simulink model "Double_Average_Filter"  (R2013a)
settings: Solver=FixedStepDiscrete  SolverMode=SingleTasking  StartTime=0.0  StopTime=inf  FixedStep=Ts  RelTol=1e-3
PreLoadFcn:
  | Implementation_Settings
StartFcn:
  | Implementation_Settings
undefined symbols (not defined in the file or in its folder): Channel, hex2dec, OffsetVolt, OutputChannel
libraries: opcode x20, pec x11

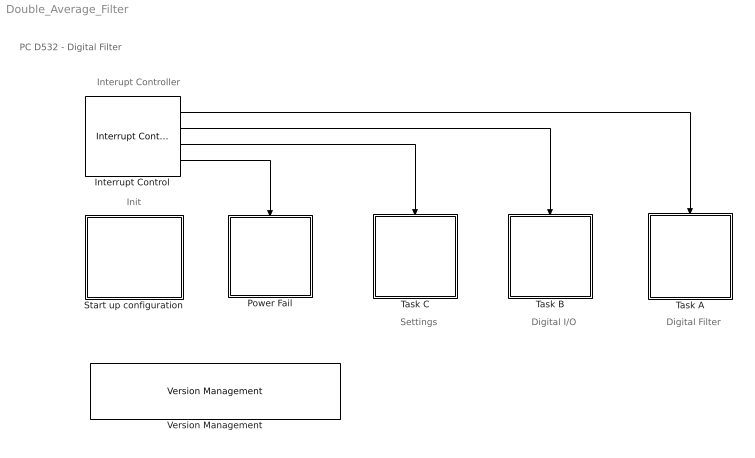
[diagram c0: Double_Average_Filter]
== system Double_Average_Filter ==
  note: PC D532 - Digital Filter
  note: Digital Filter
  note: Interupt Controller
  note: Digital I/O
  note: Settings
  note: Init
  Interrupt Control : pec/Tasks/Interrupt Control  Tag=AsyncRateTransition  EN_A=on  EN_B=on  EN_C=on  ct=Base_cycle_time  k1=Task_A_mult  k2=Task_B_mult  k3=Task_C_mult
  Power Fail : Subsystem  TreatAsAtomicUnit=on
  Start up configuration : Subsystem
  Task A : Subsystem  TreatAsAtomicUnit=on
  Task B : Subsystem  TreatAsAtomicUnit=on
  Task C : Subsystem  TreatAsAtomicUnit=on
  Version Management : pec/Logo, Info/Version Management  ApplDescr='Digital Filter'  ApplVersion='1.0.0.0'  OutPortVisible=off
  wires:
  Interrupt Control/4 -> Power Fail/Trigger
  Interrupt Control/2 -> Task B/Trigger
  Interrupt Control/3 -> Task C/Trigger
  Interrupt Control/1 -> Task A/Trigger

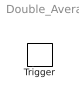
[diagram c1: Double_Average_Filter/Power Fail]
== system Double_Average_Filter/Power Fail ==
  Trigger : TriggerPort  TriggerType=function-call

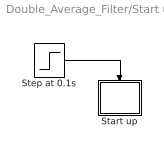
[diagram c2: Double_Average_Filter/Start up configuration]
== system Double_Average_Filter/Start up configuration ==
  Start up : Subsystem  TreatAsAtomicUnit=on
  Step at 0.1s : Step  Time=0.1  SampleTime=0
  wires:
  Step at 0.1s/1 -> Start up/Trigger

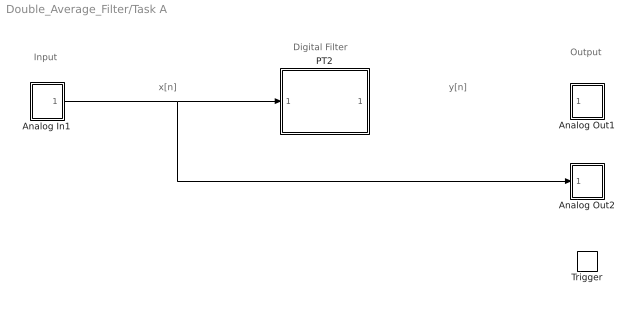
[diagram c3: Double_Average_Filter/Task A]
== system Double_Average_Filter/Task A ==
  note: Input
  note: Output
  note: Digital Filter
  note: y[n]
  note: x[n]
  Trigger : TriggerPort  TriggerType=function-call
  Analog In1 : Subsystem
  Analog Out1 : Subsystem
  Analog Out2 : Subsystem
  PT2 : Subsystem  TreatAsAtomicUnit=on
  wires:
  Analog In1/1(Out) -> PT2/1(y_in), Analog Out2/1(In1)
  ? -> Analog Out1/1(In1)

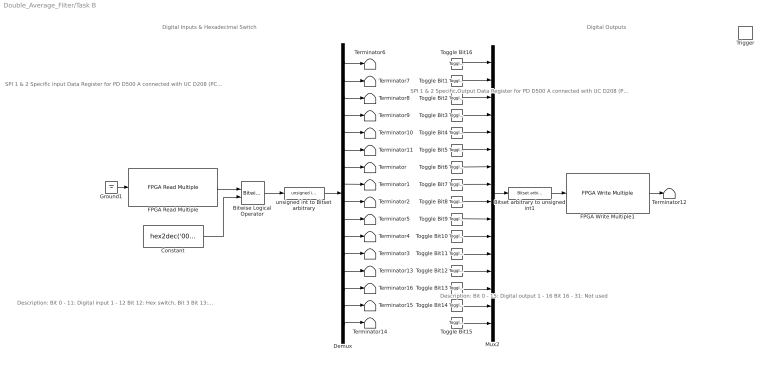
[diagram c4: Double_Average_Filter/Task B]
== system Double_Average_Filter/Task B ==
  note: Digital Inputs & Hexadecimal Switch
  note: Digital Outputs
  note: Description: Bit 0 - 15: Digital output 1 - 16 Bit 16 - 31: Not used
  note: SPI 1 & 2 Specific Output Data Register for PD D500 A connected with UC D208 (PC D532) Type: DPRAM Array 1 (32bit ports) Address offset: 0x07C000 Adress: 0x008 Mode: Write
  note: Description: Bit 0 - 11: Digital input 1 - 12 Bit 12: Hex switch, Bit 3 Bit 13: Hex switch, Bit 2 Bit 14: Hex switch, Bit 1 Bit 15: Hex switch, Bit 0 Bit 16 - 31: Not used
  note: SPI 1 & 2 Specific Input Data Register for PD D500 A connected with UC D208 (PC D532) Type: DPRAM Array 1 (32bit ports) Address offset: 0x05C000 Adress: 0x008 Mode: Read
  Trigger : TriggerPort  TriggerType=function-call
  Bitset arbitrary to unsigned int1 : opcode/Binary Signals/Bitset arbitrary to unsigned int  in_width=16  OutDataType=uint32
  Bitwise Logical Operator : pec/Math/Bitwise Logical Operator  Operator=XOR
  Constant : Constant  Value=hex2dec('00000FFF')  OutDataTypeStr=uint32
  Demux : Demux  Outputs=16
  FPGA Read Multiple : pec/Sources/FPGA Read Multiple  AddrOffsetHex=hex2dec('05c008')  number=1  datatype=uint32  pciBusPop=0  barPop=0
  FPGA Write Multiple1 : pec/Sinks/FPGA Write Multiple  AddrOffsetHex=hex2dec('07C008')  number=1  enaWriteProt=off  pciBusPop=0  barPop=0
  Ground1 : Ground
  Mux2 : Mux  Inputs=16
  Terminator{,1..16} (17 alike) : Terminator
  Toggle Bit{1..16} (16 alike) : opcode/Sources/Toggle Bit  xBit=0
  unsigned int to Bitset arbitrary : opcode/Binary Signals/unsigned int to Bitset arbitrary  InDataType=uint32  out_width=16
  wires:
  Toggle Bit2/1 -> Mux2/3
  Toggle Bit1/1 -> Mux2/2
  Toggle Bit16/1 -> Mux2/1
  Toggle Bit3/1 -> Mux2/4
  Toggle Bit4/1 -> Mux2/5
  Toggle Bit5/1 -> Mux2/6
  Toggle Bit6/1 -> Mux2/7
  Toggle Bit7/1 -> Mux2/8
  Toggle Bit8/1 -> Mux2/9
  Toggle Bit9/1 -> Mux2/10
  Toggle Bit10/1 -> Mux2/11
  Toggle Bit11/1 -> Mux2/12
  Toggle Bit12/1 -> Mux2/13
  Toggle Bit13/1 -> Mux2/14
  Toggle Bit14/1 -> Mux2/15
  Toggle Bit15/1 -> Mux2/16
  Bitset arbitrary to unsigned int1/1 -> FPGA Write Multiple1/1
  FPGA Write Multiple1/1 -> Terminator12/1
  Mux2/1 -> Bitset arbitrary to unsigned int1/1
  Demux/16 -> Terminator14/1
  Demux/15 -> Terminator15/1
  Demux/14 -> Terminator16/1
  Demux/13 -> Terminator13/1
  unsigned int to Bitset arbitrary/1 -> Demux/1
  Demux/1 -> Terminator6/1
  Demux/2 -> Terminator7/1
  Demux/3 -> Terminator8/1
  Demux/4 -> Terminator9/1
  Demux/5 -> Terminator10/1
  Demux/6 -> Terminator11/1
  Demux/7 -> Terminator/1
  Demux/8 -> Terminator1/1
  Demux/9 -> Terminator2/1
  Demux/10 -> Terminator5/1
  Demux/11 -> Terminator4/1
  Demux/12 -> Terminator3/1
  Bitwise Logical Operator/1 -> unsigned int to Bitset arbitrary/1
  Constant/1 -> Bitwise Logical Operator/2
  Ground1/1 -> FPGA Read Multiple/1
  FPGA Read Multiple/1 -> Bitwise Logical Operator/1

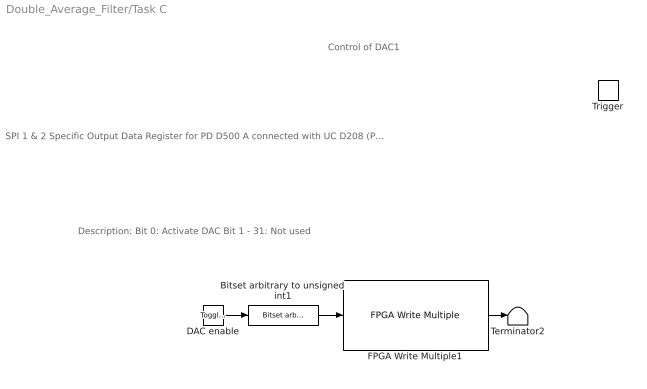
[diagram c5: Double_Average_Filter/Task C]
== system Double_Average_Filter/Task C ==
  note: SPI 1 & 2 Specific Output Data Register for PD D500 A connected with UC D208 (PC D532) Type: DPRAM Array 1 (32bit ports) Address offset: 0x07C000 Adress: 0x00C Mode: Write
  note: Description: Bit 0: Activate DAC Bit 1 - 31: Not used
  note: Control of DAC1
  Trigger : TriggerPort  TriggerType=function-call
  Bitset arbitrary to unsigned int1 : opcode/Binary Signals/Bitset arbitrary to unsigned int  in_width=1  OutDataType=uint32
  DAC enable : opcode/Sources/Toggle Bit  xBit=1
  FPGA Write Multiple1 : pec/Sinks/FPGA Write Multiple  AddrOffsetHex=hex2dec('07C00C')  number=1  enaWriteProt=off  pciBusPop=0  barPop=0
  Terminator2 : Terminator
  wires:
  Bitset arbitrary to unsigned int1/1 -> FPGA Write Multiple1/1
  DAC enable/1 -> Bitset arbitrary to unsigned int1/1
  FPGA Write Multiple1/1 -> Terminator2/1

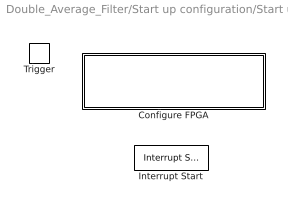
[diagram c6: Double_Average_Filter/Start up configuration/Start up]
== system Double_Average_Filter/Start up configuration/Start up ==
  Trigger : TriggerPort
  Configure FPGA : Subsystem  Priority=1
  Interrupt Start : pec/Tasks/Interrupt Start  Priority=1000

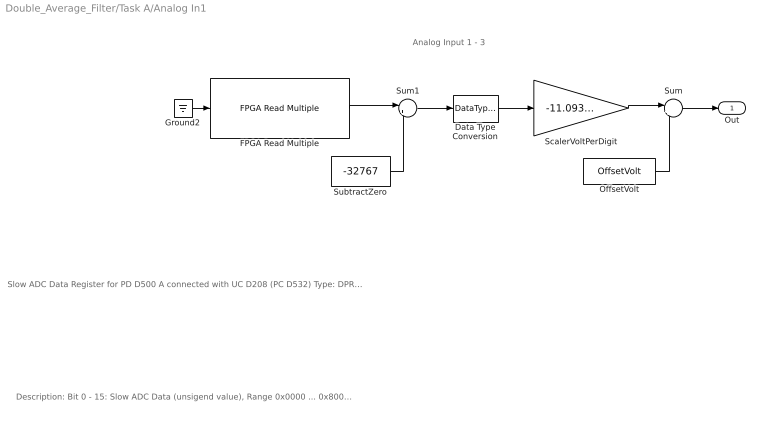
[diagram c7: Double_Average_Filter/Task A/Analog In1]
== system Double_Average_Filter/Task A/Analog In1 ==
  note: Analog Input 1 - 3
  note: Description: Bit 0 - 15: Slow ADC Data (unsigend value), Range 0x0000 ... 0x8000 ... 0xFFFF is +11.0939V ... 0 ... -11.0939V Bit 16 - 31: Not used
  note: Slow ADC Data Register for PD D500 A connected with UC D208 (PC D532) Type: DPRAM Array 1 (32bit ports) Address: 0x05C800 Address offset: 0x018 (Channel 7 - Analog Input 1) 0x01C (Channel 8 - Analog Input 2) 0x020 (Channel 9 - Analog Input 3) Mode: Read
  Data Type Conversion : DataTypeConversion  OutDataTypeStr=double
  FPGA Read Multiple : pec/Sources/FPGA Read Multiple  AddrOffsetHex=hex2dec('05c800') + 4*((Channel-1) + 6)  number=1  datatype=int32  pciBusPop=0  barPop=0
  Ground2 : Ground
  OffsetVolt : Constant  Value=OffsetVolt
  ScalerVoltPerDigit : Gain  Gain=-11.0939/32767
  SubtractZero : Constant  Value=-32767  OutDataTypeStr=int32
  Sum : Sum  Inputs=|++
  Sum1 : Sum  Inputs=|++
  Out : Outport
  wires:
  OffsetVolt/1 -> Sum/2
  Data Type Conversion/1 -> ScalerVoltPerDigit/1
  ScalerVoltPerDigit/1 -> Sum/1
  Sum/1 -> Out/1
  FPGA Read Multiple/1 -> Sum1/1
  SubtractZero/1 -> Sum1/2
  Sum1/1 -> Data Type Conversion/1
  Ground2/1 -> FPGA Read Multiple/1

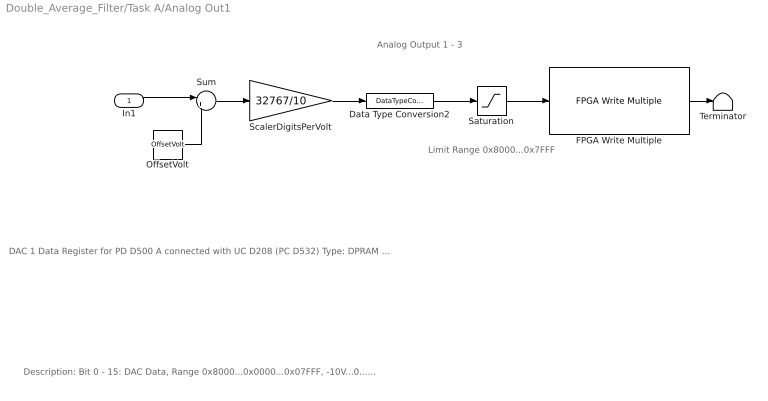
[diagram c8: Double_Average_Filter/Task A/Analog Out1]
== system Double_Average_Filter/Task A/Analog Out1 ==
  note: Limit Range 0x8000...0x7FFF
  note: DAC 1 Data Register for PD D500 A connected with UC D208 (PC D532) Type: DPRAM Array 1 (32bit ports) Address offset: 0x07C800 Adress: 0x000 (Channel 1), 0x004 (Channel 2), 0x008 (Channel 3) Mode: Write
  note: Description: Bit 0 - 15: DAC Data, Range 0x8000...0x0000...0x07FFF, -10V...0...10V, Resolution 10V/2^15 Bit 16 - 31: Not used
  note: Analog Output 1 - 3
  In1 : Inport
  Data Type Conversion2 : DataTypeConversion  OutDataTypeStr=int32
  FPGA Write Multiple : pec/Sinks/FPGA Write Multiple  AddrOffsetHex=hex2dec('07C800') + 4*(OutputChannel-1)  number=1  enaWriteProt=off  pciBusPop=0  barPop=0
  OffsetVolt : Constant  Value=OffsetVolt
  Saturation : Saturate  UpperLimit=32767  LowerLimit=-32767
  ScalerDigitsPerVolt : Gain  Gain=32767/10
  Sum : Sum  Inputs=|++
  Terminator : Terminator
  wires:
  Saturation/1 -> FPGA Write Multiple/1
  Data Type Conversion2/1 -> Saturation/1
  ScalerDigitsPerVolt/1 -> Data Type Conversion2/1
  Sum/1 -> ScalerDigitsPerVolt/1
  OffsetVolt/1 -> Sum/2
  In1/1 -> Sum/1
  FPGA Write Multiple/1 -> Terminator/1

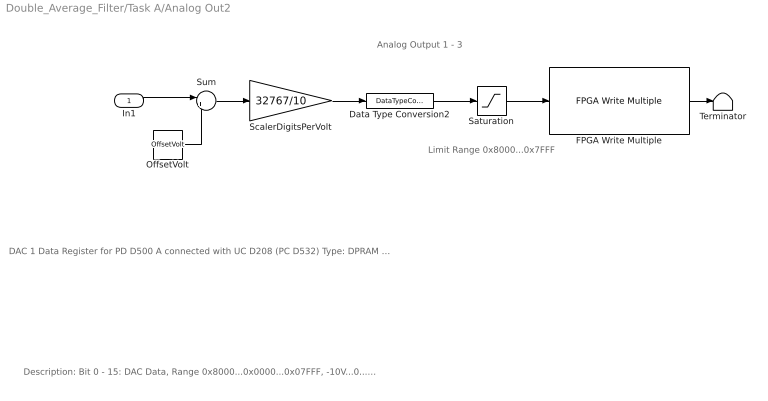
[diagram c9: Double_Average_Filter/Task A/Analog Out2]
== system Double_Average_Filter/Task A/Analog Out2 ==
  note: Analog Output 1 - 3
  note: Description: Bit 0 - 15: DAC Data, Range 0x8000...0x0000...0x07FFF, -10V...0...10V, Resolution 10V/2^15 Bit 16 - 31: Not used
  note: DAC 1 Data Register for PD D500 A connected with UC D208 (PC D532) Type: DPRAM Array 1 (32bit ports) Address offset: 0x07C800 Adress: 0x000 (Channel 1), 0x004 (Channel 2), 0x008 (Channel 3) Mode: Write
  note: Limit Range 0x8000...0x7FFF
  In1 : Inport
  Data Type Conversion2 : DataTypeConversion  OutDataTypeStr=int32
  FPGA Write Multiple : pec/Sinks/FPGA Write Multiple  AddrOffsetHex=hex2dec('07C800') + 4*(OutputChannel-1)  number=1  enaWriteProt=off  pciBusPop=0  barPop=0
  OffsetVolt : Constant  Value=OffsetVolt
  Saturation : Saturate  UpperLimit=32767  LowerLimit=-32767
  ScalerDigitsPerVolt : Gain  Gain=32767/10
  Sum : Sum  Inputs=|++
  Terminator : Terminator
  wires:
  FPGA Write Multiple/1 -> Terminator/1
  In1/1 -> Sum/1
  OffsetVolt/1 -> Sum/2
  Sum/1 -> ScalerDigitsPerVolt/1
  ScalerDigitsPerVolt/1 -> Data Type Conversion2/1
  Data Type Conversion2/1 -> Saturation/1
  Saturation/1 -> FPGA Write Multiple/1

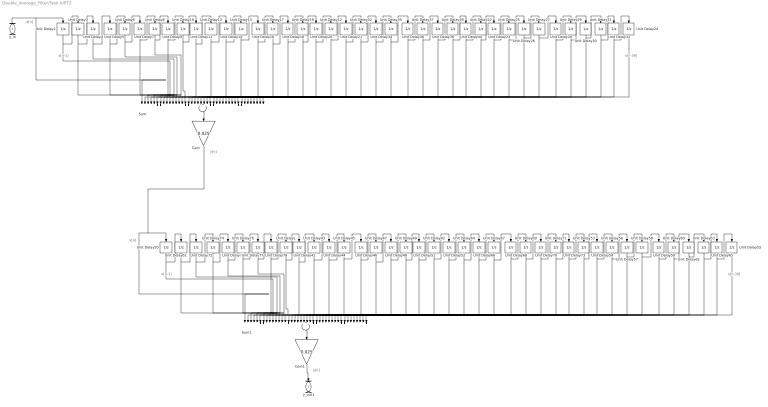
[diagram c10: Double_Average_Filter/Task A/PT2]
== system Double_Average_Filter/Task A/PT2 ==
  note: x[n]
  note: x[n-39]
  note: y[n]
  note: x[n-1]
  note: x[n]
  note: x[n-39]
  note: y[n]
  note: x[n-1]
  y_in : Inport
  Gain : Gain  Gain=0.025
  Gain1 : Gain  Gain=0.025
  Sum : Sum  Inputs=++++++++++++++++++++++++++++++++++++++++
  Sum1 : Sum  Inputs=++++++++++++++++++++++++++++++++++++++++
  Unit Delay{1..78} (78 alike) : UnitDelay  SampleTime=-1
  y_out1 : Outport
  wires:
  Sum/1 -> Gain/1
  Unit Delay2/1 -> Sum/2, Unit Delay3/1
  Unit Delay3/1 -> Sum/3, Unit Delay4/1
  Unit Delay4/1 -> Sum/4, Unit Delay5/1
  Unit Delay5/1 -> Sum/5, Unit Delay6/1
  Unit Delay6/1 -> Sum/6, Unit Delay7/1
  Unit Delay7/1 -> Sum/7, Unit Delay8/1
  Unit Delay8/1 -> Sum/8, Unit Delay9/1
  Unit Delay9/1 -> Sum/9, Unit Delay10/1
  Unit Delay10/1 -> Sum/10, Unit Delay11/1
  Unit Delay11/1 -> Sum/11, Unit Delay13/1
  Unit Delay13/1 -> Sum/12, Unit Delay14/1
  Unit Delay14/1 -> Sum/13, Unit Delay15/1
  Unit Delay15/1 -> Sum/14, Unit Delay16/1
  Unit Delay16/1 -> Sum/15, Unit Delay17/1
  Unit Delay17/1 -> Sum/16, Unit Delay18/1
  Unit Delay18/1 -> Sum/17, Unit Delay19/1
  Unit Delay19/1 -> Sum/18, Unit Delay20/1
  Unit Delay20/1 -> Sum/19, Unit Delay12/1
  Unit Delay12/1 -> Sum/20, Unit Delay21/1
  Unit Delay21/1 -> Sum/21, Unit Delay32/1
  Unit Delay32/1 -> Sum/22, Unit Delay34/1
  Unit Delay34/1 -> Sum/23, Unit Delay35/1
  Unit Delay35/1 -> Sum/24, Unit Delay36/1
  Unit Delay36/1 -> Sum/25, Unit Delay37/1
  Unit Delay37/1 -> Sum/26, Unit Delay38/1
  Unit Delay38/1 -> Sum/27, Unit Delay39/1
  Unit Delay39/1 -> Sum/28, Unit Delay40/1
  Unit Delay40/1 -> Sum/29, Unit Delay22/1
  Unit Delay22/1 -> Sum/30, Unit Delay23/1
  Unit Delay23/1 -> Sum/31, Unit Delay25/1
  Unit Delay25/1 -> Sum/32, Unit Delay26/1
  Unit Delay26/1 -> Sum/33, Unit Delay27/1
  Unit Delay27/1 -> Sum/34, Unit Delay28/1
  Unit Delay28/1 -> Sum/35, Unit Delay29/1
  Unit Delay29/1 -> Sum/36, Unit Delay30/1
  Unit Delay30/1 -> Sum/37, Unit Delay31/1
  Unit Delay31/1 -> Sum/38, Unit Delay33/1
  Unit Delay33/1 -> Sum/39, Unit Delay24/1
  Unit Delay24/1 -> Sum/40
  y_in/1 -> Unit Delay2/1, Sum/1
  Gain1/1 -> y_out1/1
  Sum1/1 -> Gain1/1
  Unit Delay50/1 -> Sum1/2, Unit Delay61/1
  Unit Delay61/1 -> Sum1/3, Unit Delay72/1
  Unit Delay72/1 -> Sum1/4, Unit Delay74/1
  Unit Delay74/1 -> Sum1/5, Unit Delay75/1
  Unit Delay75/1 -> Sum1/6, Unit Delay76/1
  Unit Delay76/1 -> Sum1/7, Unit Delay77/1
  Unit Delay77/1 -> Sum1/8, Unit Delay78/1
  Unit Delay78/1 -> Sum1/9, Unit Delay1/1
  Unit Delay1/1 -> Sum1/10, Unit Delay41/1
  Unit Delay41/1 -> Sum1/11, Unit Delay43/1
  Unit Delay43/1 -> Sum1/12, Unit Delay44/1
  Unit Delay44/1 -> Sum1/13, Unit Delay45/1
  Unit Delay45/1 -> Sum1/14, Unit Delay46/1
  Unit Delay46/1 -> Sum1/15, Unit Delay47/1
  Unit Delay47/1 -> Sum1/16, Unit Delay48/1
  Unit Delay48/1 -> Sum1/17, Unit Delay49/1
  Unit Delay49/1 -> Sum1/18, Unit Delay51/1
  Unit Delay51/1 -> Sum1/19, Unit Delay42/1
  Unit Delay42/1 -> Sum1/20, Unit Delay52/1
  Unit Delay52/1 -> Sum1/21, Unit Delay64/1
  Unit Delay64/1 -> Sum1/22, Unit Delay66/1
  Unit Delay66/1 -> Sum1/23, Unit Delay67/1
  Unit Delay67/1 -> Sum1/24, Unit Delay68/1
  Unit Delay68/1 -> Sum1/25, Unit Delay69/1
  Unit Delay69/1 -> Sum1/26, Unit Delay70/1
  Unit Delay70/1 -> Sum1/27, Unit Delay71/1
  Unit Delay71/1 -> Sum1/28, Unit Delay73/1
  Unit Delay73/1 -> Sum1/29, Unit Delay53/1
  Unit Delay53/1 -> Sum1/30, Unit Delay54/1
  Unit Delay54/1 -> Sum1/31, Unit Delay56/1
  Unit Delay56/1 -> Sum1/32, Unit Delay57/1
  Unit Delay57/1 -> Sum1/33, Unit Delay58/1
  Unit Delay58/1 -> Sum1/34, Unit Delay59/1
  Unit Delay59/1 -> Sum1/35, Unit Delay60/1
  Unit Delay60/1 -> Sum1/36, Unit Delay62/1
  Unit Delay62/1 -> Sum1/37, Unit Delay63/1
  Unit Delay63/1 -> Sum1/38, Unit Delay65/1
  Unit Delay65/1 -> Sum1/39, Unit Delay55/1
  Unit Delay55/1 -> Sum1/40
  Gain/1 -> Sum1/1, Unit Delay50/1

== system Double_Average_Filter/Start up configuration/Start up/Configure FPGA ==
  For Iterator Subsystem : Subsystem  TreatAsAtomicUnit=on

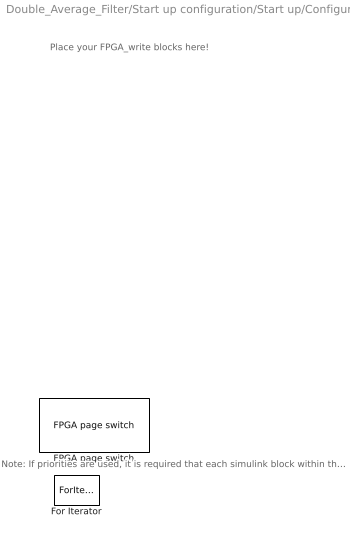
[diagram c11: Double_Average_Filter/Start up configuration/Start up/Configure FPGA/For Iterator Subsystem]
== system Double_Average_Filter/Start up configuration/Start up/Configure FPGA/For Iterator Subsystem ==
  note: Place your FPGA_write blocks here!
  note: Note: If priorities are used, it is required that each simulink block within this 'for iterator subsystem' has a priority and that the blocks 'FPGA page switch' and 'For Iterator' have the lowest one.
  FPGA page switch : pec/Sources/FPGA page switch
  For Iterator : ForIterator  IterationLimit=2  ShowIterationPort=off
